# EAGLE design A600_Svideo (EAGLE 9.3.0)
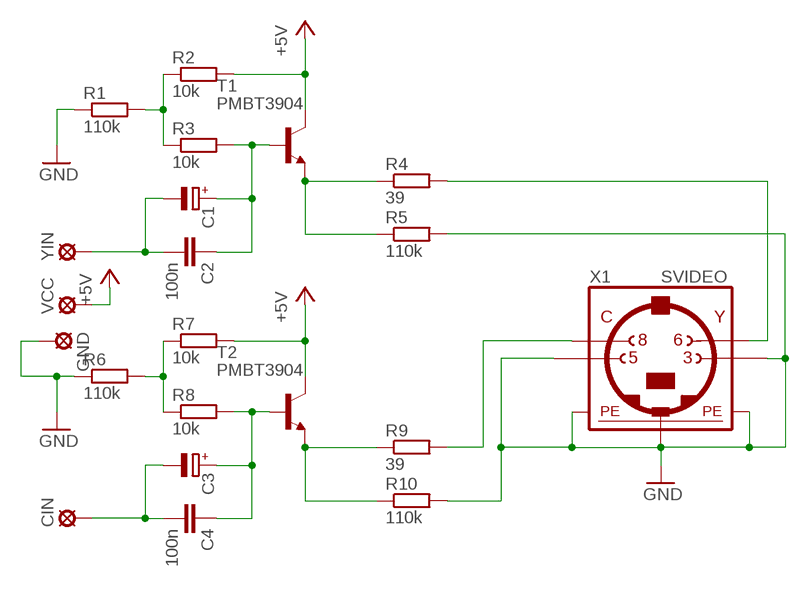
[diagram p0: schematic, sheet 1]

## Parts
C1  CPOL-EUSMCC  [SMC_C]
C2  100n  C-EUC0805  [C0805]
C3  CPOL-EUSMCC  [SMC_C]
C4  100n  C-EUC0805K  [C0805K]
CIN  LSP11  [LSP11]
GND  LSP11  [LSP11]
R1  110k  R-EU_M0805  [M0805]
R2  10k  R-EU_M0805  [M0805]
R3  10k  R-EU_M0805  [M0805]
R4  39  R-EU_M0805  [M0805]
R5  110k  R-EU_M0805  [M0805]
R6  110k  R-EU_M0805  [M0805]
R7  10k  R-EU_M0805  [M0805]
R8  10k  R-EU_M0805  [M0805]
R9  39  R-EU_M0805  [M0805]
R10  110k  R-EU_M0805  [M0805]
T1  PMBT3904  BC847B-NPN-SOT23-BEC  [SOT23-BEC]
T2  PMBT3904  BC847B-NPN-SOT23-BEC  [SOT23-BEC]
VCC  LSP11  [LSP11]
X1  SVIDEO  MINI_DIN_4  [M_DIN4]
YIN  LSP11  [LSP11]

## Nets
+5V: R2.2 R7.2 T1.C T2.C VCC.MP
CROMA: R9.2 X1.8
GND: GND.MP R1.1 R5.2 R6.1 R10.2 X1.3 X1.5 X1.SH1(PE1) X1.SH2(PE2) X1.SH3(PE3)
LUMA: R4.2 X1.6
N$1: C1.- C2.2 YIN.MP
N$2: C1.+ C2.1 R3.2 T1.B
N$3: R1.2 R2.1 R3.1
N$4: R4.1 R5.1 T1.E
N$5: C3.- C4.2 CIN.MP
N$7: C3.+ C4.1 R8.2 T2.B
N$8: R6.2 R7.1 R8.1
N$9: R9.1 R10.1 T2.E

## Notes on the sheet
- C | Y

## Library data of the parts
C1 C3 = rcl:CPOL-EU: POLARIZED CAPACITOR, European symbol
C2 C4 = rcl:C-EU: CAPACITOR, European symbol
CIN GND VCC YIN = solpad:LSP11: SOLDER PAD
R1-R10 = rcl:R-EU_: RESISTOR, European symbol
T1 T2 = transistor:*-NPN-: NPN Transistror BF959 corrected 2008.03.06
X1 = mini_din:MINI_DIN_4

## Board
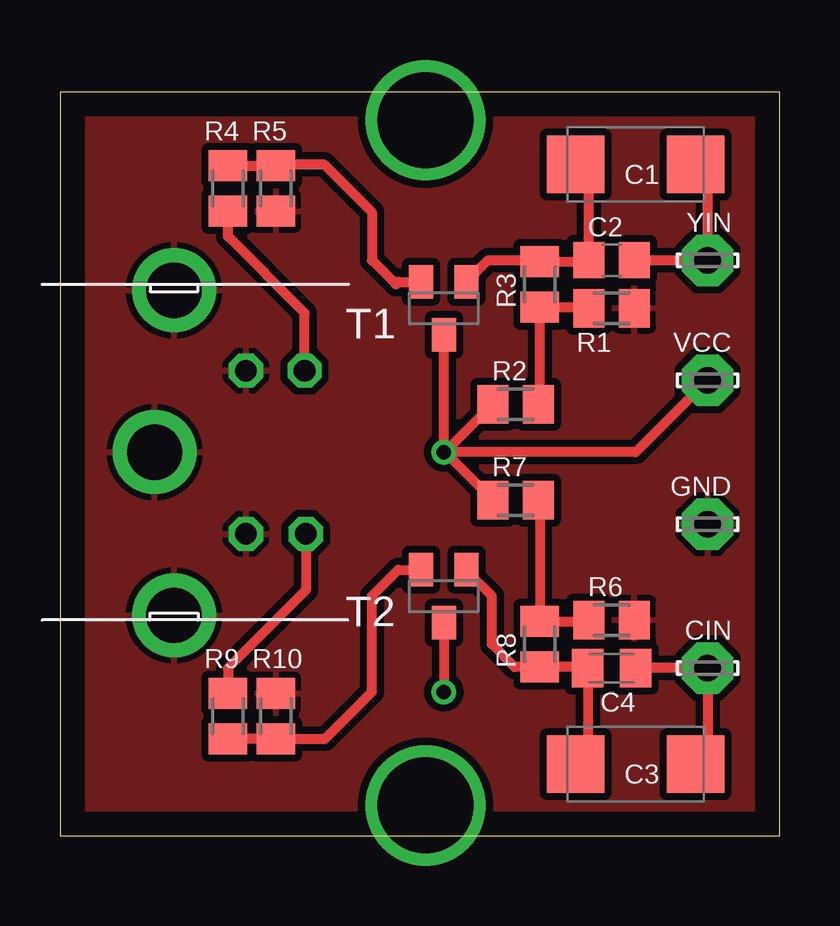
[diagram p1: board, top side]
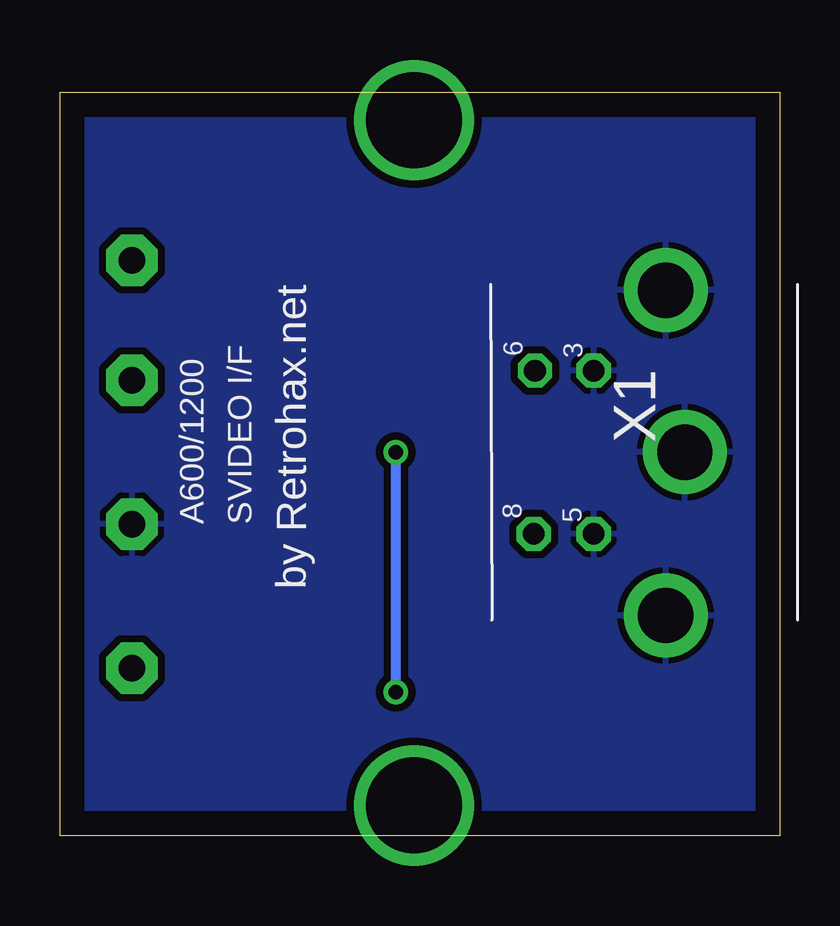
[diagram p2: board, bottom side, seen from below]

Size 30 x 31 mm. Coordinates in mm from the lower left corner, seen from the top.
Outline: 0,0 30,0 30,31 0,31 0,0
Copper layers (1*16): Top 0.035mm / dielectric 1.5mm / Bottom 0.035mm
Design rules "default *": minimum track width 10mil, minimum drill 24mil, track to track 12mil, track to pad 12mil, pad to pad 12mil, via to via 12mil, smd to smd 12mil, copper to edge 40mil, drill to drill 8mil, minimum pad ring 10mil, minimum via ring 8mil, stop-mask expansion 4mil, vias tented up to drill 0mil, thermal gap 10mil

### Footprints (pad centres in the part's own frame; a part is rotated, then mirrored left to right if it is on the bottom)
SMC_C = smd 2.4 x 2.4: + -2.5,0; - 2.5,0
C0805 = smd 1.3 x 1.5: 1 -0.95,0; 2 0.95,0
C0805K = smd 1.3 x 1.6: 1 -1,0; 2 1,0
LSP11 = drill 1.118 pad 2.159 octagon: MP 0,0
M0805 = smd 1.3 x 1.6: 1 -0.95,0; 2 0.95,0
SOT23-BEC = smd 1 x 1.4: B -0.95,-1.1; C 0,1.1; E 0.95,-1.1
M_DIN4 = drill 0.9 pad 1.422 octagon: 3 -3.4,-3.75; 5 3.4,-3.75; 6 -3.4,-6.2; 8 3.4,-6.25 | drill 2.3 pad 3.5: SH1 6.8,-0.75; SH2 0,0.05; SH3 -6.75,-0.75

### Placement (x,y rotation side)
C1  24,28 0 top
C2  23,24 0 top
C3  24,3 0 top
C4  23,7 0 top
CIN  27,7 0 top
GND  27,13 0 top
R1  23,22 180 top
R2  19,18 180 top
R3  20,23 90 top
R4  7,27 270 top
R5  9,27 270 top
R6  23,9 180 top
R7  19,14 180 top
R8  20,8 270 top
R9  7,5 90 top
R10  9,5 90 top
T1  16,22 180 top
T2  16,10 180 top
VCC  27,19 0 top
X1  4,16 270 bottom
YIN  27,24 0 top

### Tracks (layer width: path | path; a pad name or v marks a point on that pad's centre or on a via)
+5V  (via drill 0.61)
  Top 0.406: VCC.MP 24,16 16.05,16 | T2.C v16,6 | 16.05,16 R2.2 | 16.05,16 v16,16 T1.C | 16.05,16 R7.2
  Bottom 0.406: v16,6 v16,16
CROMA
  Top 0.406: X1.8 10.25,10.25 7,7 R9.2
GND
  pour Top: 0,31 30,31 30,0 0,0
  pour Bottom: 0,0 30,0 30,31 0,31
LUMA
  Top 0.406: X1.6 10.2,21.8 7,25 R4.2
N$1
  Top 0.406: C2.2 YIN.MP 27,27.5 C1.-
N$2
  Top 0.406: T1.B 17.85,24 19.95,24 R3.2 22,23.95 C2.1 22.05,27.45 C1.+
N$3
  Top 0.406: R2.1 20,18.05 R3.1 22,22.05 R1.2
N$4
  Top 0.406: R4.1 R5.1 9.05,28 11,28 13,26 13,24 14,23 14.1,23.1 T1.E
N$5
  Top 0.406: C4.2 CIN.MP 27,3.5 C3.-
N$6  (via drill 4)
  other vias: 15.24,1.27
N$7
  Top 0.406: T2.B 16.95,11.05 18,10 18,8 18.95,7.05 R8.2 21.95,7.05 C4.1 22,3.5 C3.+
N$8
  Top 0.406: R7.1 20,13.95 R8.1 22,8.95 R6.2
N$9
  Top 0.406: R9.1 R10.1 11.05,4.05 13,6 13,10 14.1,11.1 T2.E
N$10  (via drill 4)
  other vias: 15.24,29.84

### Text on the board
bPlace: by Retrohax.net | SVIDEO I/F | A600/1200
